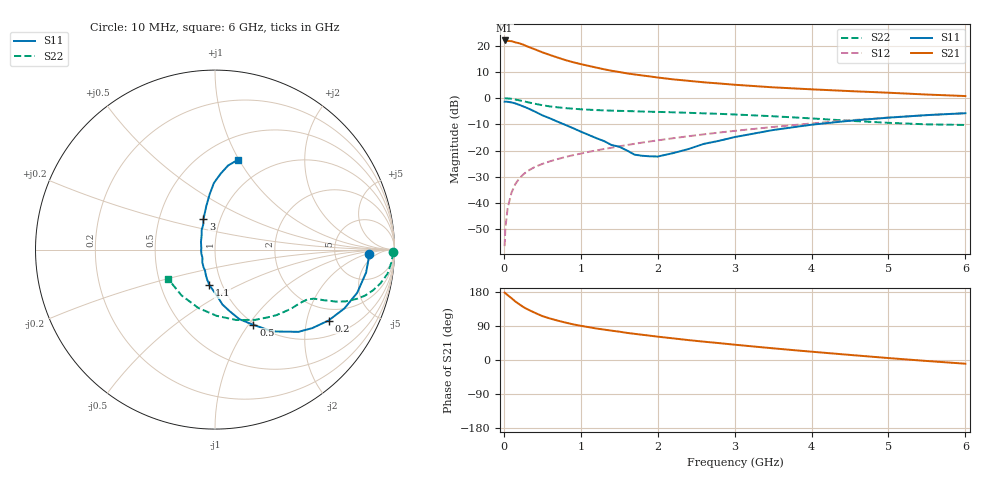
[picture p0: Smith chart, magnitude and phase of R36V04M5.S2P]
! SIEMENS Small Signal Semiconductors
! BFR181
! Si NPN RF Bipolar Junction Transistor in SOT23
! VCE = 6 V  IC = 4.5 mA
! Common Emitter S-Parameters:  May  1996
# GHz  S  MA  R  50
!  f  S11  S21  S12  S22
! GHz  MAG  ANG  MAG  ANG  MAG  ANG  MAG  ANG
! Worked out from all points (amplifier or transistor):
!   36 points, 10 MHz to 6 GHz, reference 50 ohm
!   highest |S21| = 22.0 dB at 10 MHz (marker M1)
!   |S21| within 3 dB of that: start of sweep to 369.4 MHz
!   unconditionally stable (mu >= 1): 1.218 GHz to 3.073 GHz
!   at 250 MHz: K = 0.39, MSG = 24.8 dB, |S12| = -29.2 dB
!   at 1.4 GHz: K = 1.04, MAG = 13.5 dB, |S12| = -18.9 dB
!   at 6 GHz: K = 0.86, MSG = 3.3 dB, |S12| = -5.7 dB
!   S11 on the Smith chart (normalised r, x): 10 MHz: 13, -3; 200 MHz: 1.52, -2.71; 500 MHz: 0.98, -1.06; 1.1 GHz: 0.87, -0.36; 3 GHz: 0.83, +0.29; 6 GHz: 0.73, +0.99
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0.01  0.8585 -1.8  12.59 177.9  0.0015 96.6  0.9931 -0.8
0.02  0.8576 -3.3  12.29 176.1  0.0033 85.2  0.9915 -1.7
0.05  0.8516 -8.6  12.37 171.2  0.0081 86.1  0.9857 -4.1
0.1  0.8279 -16.9  12.19 163.0  0.0158 81.6  0.9705 -8.0
0.15  0.7917 -24.5  11.57 154.4  0.023 76.7  0.9405 -11.6
0.2  0.7457 -32.0  11.13 147.2  0.0293 73.9  0.9085 -14.5
0.25  0.6966 -38.9  10.51 140.3  0.0347 69.8  0.875 -17.0
0.3  0.6526 -44.6  9.746 134.5  0.04 68.3  0.8416 -18.9
0.4  0.5572 -54.9  8.569 124.9  0.0484 65.4  0.7836 -21.6
0.5  0.4703 -63.0  7.484 115.9  0.0556 63.5  0.7324 -23.3
0.6  0.4113 -70.6  6.642 109.5  0.0624 62.5  0.6936 -24.2
0.8  0.3086 -82.3  5.317 98.8  0.0754 62.3  0.6447 -25.5
0.9  0.2673 -86.3  4.844 94.1  0.0816 62.4  0.6281 -26.0
1.1  0.1996 -99.0  4.128 86.8  0.0942 63.0  0.6019 -27.2
1.3  0.1522 -109.4  3.557 80.3  0.107 63.3  0.5837 -28.5
1.6  0.1003 -134.7  2.968 71.6  0.1274 63.2  0.5664 -31.0
2.2  0.0893 151.1  2.28 57.1  0.1718 61.9  0.5365 -37.9
3  0.1807 110.9  1.8 40.4  0.2375 57.5  0.4879 -49.9
3.5  0.2463 101.4  1.606 30.8  0.2818 53.7  0.4511 -60.2
4.5  0.3704 91.0  1.361 13.4  0.3781 43.9  0.3693 -88.5
5.5  0.4746 81.1  1.17 -2.6  0.4735 31.6  0.316 -126.3
6  0.5152 75.8  1.096 -9.8  0.5175 24.6  0.3077 -147.5
